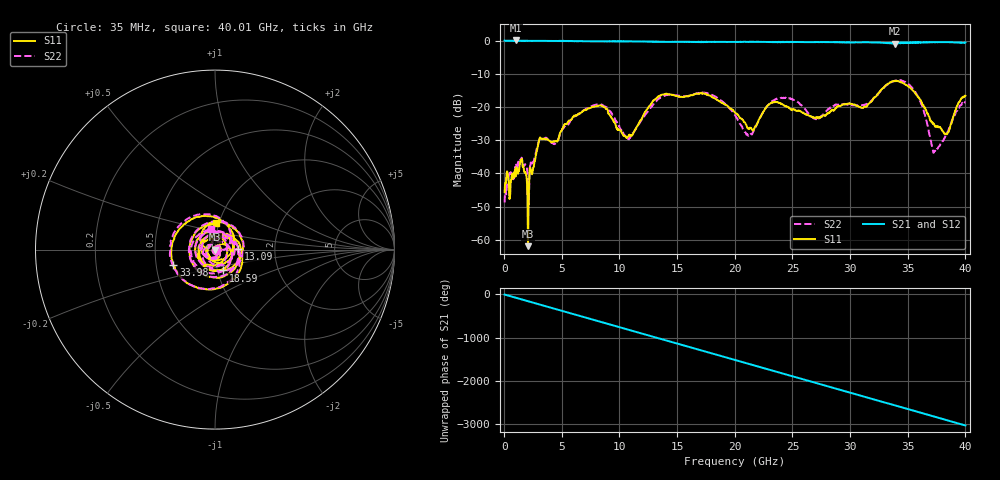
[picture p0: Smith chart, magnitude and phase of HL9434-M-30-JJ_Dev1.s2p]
! 5/27/2020 7:35:46 AM
! H:\PRODUCTION_DATA\TEMP_S2P.S2P
! CHANNEL.1
! TR.MEASUREMENT
! CORRECTED.DATA
# GHZ S RI R 50.0
! FREQ.GHZ  S11RE  S11IM  S21RE  S21IM  S12RE  S12IM  S22RE  S22IM
!; PortSelection: Port_12
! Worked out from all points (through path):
!   1143 points, 35 MHz to 40.01 GHz, reference 50 ohm
!   highest |S21| = 0.04 dB at 1.05 GHz (marker M1); lowest = -0.9 dB at 33.91 GHz (marker M2)
!   group delay of S21, straight-line fit = 210 ps
!   lowest |S11| = -61.9 dB at 2.065 GHz (marker M3), VSWR 1.00, Z = 50.1 - j0.0336 ohm
!   |S11| at or under -10 dB: start of sweep to end of sweep
!   |S22| runs from -49.4 to -11.9 dB; largest |S21 - S12| = 0.037
!   S11 on the Smith chart (normalised r, x): 35 MHz: 1.01, -0.01; 13.09 GHz: 1.30, +0.02; 18.59 GHz: 1.06, -0.25; 33.98 GHz: 0.62, -0.11; 40.01 GHz: 0.96, +0.29
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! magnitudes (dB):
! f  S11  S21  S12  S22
! 35 MHz  -45.6  0.0  0.0  -48.7
! 1.05 GHz  -38.1  0.0  0.0  -37.3
! 1.54 GHz  -35.6  -0.1  -0.1  -35.4
! 2.065 GHz  -61.9  -0.1  -0.1  -43.1
! 3.115 GHz  -29.2  -0.1  -0.1  -29.4
! 6.72 GHz  -21.6  -0.2  -0.2  -21.5
! 8.61 GHz  -19.9  -0.2  -0.2  -19.6
! 10.64 GHz  -29.4  -0.2  -0.2  -29.4
! 13.09 GHz  -17.7  -0.3  -0.3  -18.7
! 13.37 GHz  -16.9  -0.4  -0.3  -17.6
! 18.59 GHz  -18.1  -0.4  -0.4  -17.5
! 20.02 GHz  -21.7  -0.4  -0.4  -22.5
! 21.18 GHz  -26.5  -0.4  -0.4  -28.7
! 23.7 GHz  -18.5  -0.4  -0.5  -17.4
! 26.7 GHz  -23.0  -0.4  -0.4  -23.0
! 33.35 GHz  -12.9  -0.8  -0.7  -13.0
! 33.91 GHz  -12.1  -0.9  -0.7  -12.1
! 33.98 GHz  -12.2  -0.7  -0.7  -12.0
! 35.77 GHz  -16.4  -0.5  -0.7  -16.1
! 37.34 GHz  -25.7  -0.5  -0.5  -33.3
! 38.4 GHz  -28.2  -0.5  -0.5  -28.1
! 40.01 GHz  -16.6  -0.6  -0.6  -18.6
